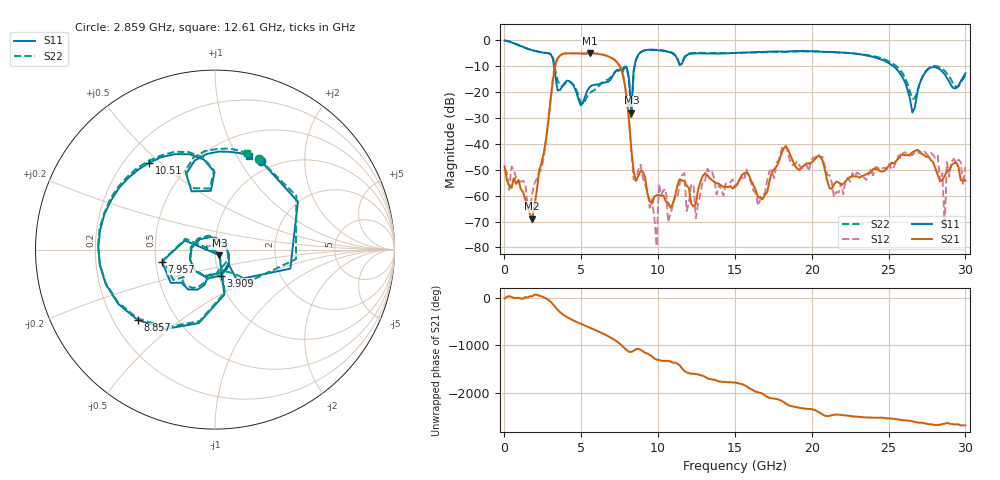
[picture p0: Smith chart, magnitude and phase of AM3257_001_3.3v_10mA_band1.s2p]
!Keysight Technologies,N5245B,MY58422270,A.16.20.02
!Date: Wednesday, June 18, 2025 21:01:45
!Correction: S11(C  2-Port  )
!S21(C  2-Port  )
!S12(C  2-Port  )
!S22(C  2-Port  )
!S2P File: Measurements: S11, S21, S12, S22:
# Hz S  dB  R 50
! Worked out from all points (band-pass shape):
!   201 points, 10 MHz to 30 GHz, reference 50 ohm
!   highest |S21| = -5.09 dB at 5.558 GHz (marker M1); lowest = -68.8 dB at 1.809 GHz (marker M2)
!   |S21| within 3 dB of the highest: 3.405 GHz to 7.245 GHz (3.84 GHz wide, 72.1 % of centre)
!   lowest |S11| = -28.0 dB at 8.257 GHz (marker M3), VSWR 1.08, Z = 52.4 - j3.28 ohm
!   |S11| at or under -10 dB: 3.223 GHz to 8.471 GHz (5.248 GHz wide, 89.8 % of centre); 25.29 GHz to end of sweep
!   |S22| runs from -29.8 to -0.1 dB; largest |S21 - S12| = 0.048
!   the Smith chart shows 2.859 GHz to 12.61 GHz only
!   S11 on the Smith chart (normalised r, x): 2.859 GHz: 0.87, +1.24; 3.909 GHz: 1.02, -0.30; 7.957 GHz: 0.54, -0.08; 8.857 GHz: 0.30, -0.36; 10.51 GHz: 0.30, +0.46; 12.61 GHz: 0.75, +1.13
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1e7  -0.16 -1.8  -48.70 -18.9  -49.59 -81.4  -0.14 -1.0
7.5975e8  -1.56 -86.8  -55.46 -10.4  -53.37 -49.2  -1.56 -86.5
1.8094e9  -3.92 -179.2  -68.83 26.1  -59.05 51.0  -3.90 -179.4
2.85905e9  -5.10 62.4  -30.89 -50.2  -31.39 -47.3  -5.00 64.1
3.9087e9  -16.57 -77.6  -5.22 -19.1  -5.16 -20.2  -17.08 -87.9
5.1083e9  -24.24 16.2  -5.20 146.3  -5.24 146.2  -24.83 39.7
5.55815e9  -18.07 -64.6  -5.09 84.8  -5.07 84.9  -20.44 -50.7
7.95735e9  -10.36 -167.2  -22.54 -28.2  -21.72 -31.4  -10.65 -168.8
8.25725e9  -28.01 -51.7  -42.19 -66.3  -42.76 -88.9  -29.78 -39.6
8.85705e9  -4.70 -137.5  -50.46 -20.5  -48.08 -4.9  -4.78 -138.3
9.9067e9  -3.87 154.8  -59.87 133.1  -79.50 -134.4  -3.76 154.2
1.005665e10  -3.93 147.5  -59.77 125.0  -55.44 58.4  -3.85 146.9
1.05065e10  -4.34 127.0  -62.22 107.5  -57.59 109.3  -4.20 126.7
1.26058e10  -5.10 69.9  -57.62 179.8  -62.89 -162.8  -4.93 71.4
1.5005e10  -4.99 -4.0  -56.55 8.4  -56.82 26.5  -4.96 -0.4
2.01033e10  -4.27 -105.6  -46.60 158.1  -45.28 151.9  -4.42 -104.8
2.505165e10  -9.00 170.3  -48.53 -27.3  -47.68 -25.4  -8.31 173.6
2.655115e10  -27.97 -174.4  -43.25 -84.9  -44.30 -77.6  -22.66 -177.0
2.82006e10  -10.89 -150.4  -52.03 -161.0  -44.56 -174.3  -10.16 -155.4
2.865045e10  -13.17 -162.2  -52.47 -137.1  -72.50 -124.5  -11.86 -167.5
2.88004e10  -14.57 -163.7  -50.40 -121.9  -47.05 -126.7  -12.88 -169.2
3e10  -12.80 -94.2  -54.21 -171.4  -48.98 -107.2  -13.43 -100.5
